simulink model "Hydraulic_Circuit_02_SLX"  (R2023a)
settings: Solver=ode23s  StartTime=0.0  StopTime=10.0  MaxStep=0.001  RelTol=1e-3
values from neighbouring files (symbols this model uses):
  C_5 = 0.001*m^3/Pa    (= 0.001)    [Hydraulic_Circuit_02_EQN.m]    (also in Hydraulic_Circuit_02_SLX_m.m; Electric_Circuit_02_EQN.m; Electric_Circuit_02_SLX_m.m; Electric_Circuit_04_EQN.m)
  C_7 = 0.001*m^3/Pa    (= 0.001)    [Hydraulic_Circuit_02_EQN.m]    (also in Hydraulic_Circuit_02_SLX_m.m; Electric_Circuit_02_EQN.m; Electric_Circuit_02_SLX_m.m; Electric_Circuit_04_EQN.m)
  L_4 = 10*Pa*sec^2/m^3    (= 10)    [Hydraulic_Circuit_02_EQN.m]    (also in Hydraulic_Circuit_02_SLX_m.m; Electric_Circuit_02_EQN.m = 0.002; Electric_Circuit_02_SLX_m.m = 0.002; Electric_Circuit_03_EQN.m = 0.002)
  L_6 = 10*Pa*sec^2/m^3    (= 10)    [Hydraulic_Circuit_02_EQN.m]    (also in Hydraulic_Circuit_02_SLX_m.m; Electric_Circuit_07_EQN.m = 0.002; Electric_Circuit_07_SLX_m.m = 0.002; Hydraulic_Circuit_03_EQN.m)
  P_1_0 = 10*Pa    (= 10)    [Hydraulic_Circuit_02_SLX_m.m]    (also in Hydraulic_Circuit_01_SLX_m.m; Hydraulic_Circuit_03_SLX_m.m; Hydraulic_Clutch_System_SLX_m.m)
  P_5_0 = 0*Pa    (= 0)    [Hydraulic_Circuit_02_SLX_m.m]    (also in Hydraulic_Circuit_03_SLX_m.m)
  P_7_0 = 0*Pa    (= 0)    [Hydraulic_Circuit_02_SLX_m.m]
  Q_4_0 = 0*m^3/sec    (= 0)    [Hydraulic_Circuit_02_SLX_m.m]    (also in Hydraulic_Circuit_03_SLX_m.m)
  Q_6_0 = 0*m^3/sec    (= 0)    [Hydraulic_Circuit_02_SLX_m.m]    (also in Hydraulic_Circuit_03_SLX_m.m)
  Q_9_0 = 0*m^3/sec    (= 0)    [Hydraulic_Circuit_02_SLX_m.m]
  R_2 = 10000*Pa/(m^3/sec)    (= 10000)    [Hydraulic_Circuit_02_EQN.m]    (also in Hydraulic_Circuit_02_SLX_m.m; BIG_EC_Simscape_EQN.m = 100; BIG_EC_Simscape_SLX_m.m = 100; Electric_Circuit_07_EQN.m = 100)
  R_3 = 10000*Pa/(m^3/sec)    (= 10000)    [Hydraulic_Circuit_02_EQN.m]    (also in Hydraulic_Circuit_02_SLX_m.m; Electric_Circuit_01_EQN.m = 100; Electric_Circuit_01_SLX_m.m = 100; Electric_Circuit_02_EQN.m = 100)
  R_8 = 10000*Pa/(m^3/sec)    (= 10000)    [Hydraulic_Circuit_02_EQN.m]    (also in Hydraulic_Circuit_02_SLX_m.m; Electric_Circuit_10_EQN.m = 100; Electric_Circuit_10_SLX_m.m = 100)
  Ts = Tfin/Nr_Ts_Points    (= 0.03999985)    [Hydraulic_Circuit_02_SLX_m.m]    (also in BIG_EC_Simscape_SLX_m.m = 0.0003; Car_Dumper_SLX_m.m = 0.0022779; Electric_Circuit_01_SLX_m.m = 0.005; Electric_Circuit_02_SLX_m.m = 0.000480145)

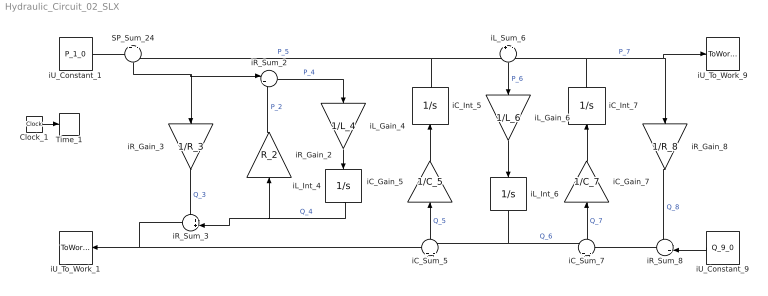
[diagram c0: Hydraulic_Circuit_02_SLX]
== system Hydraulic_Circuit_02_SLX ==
  Clock_1 : Clock
  SP_Sum_24 : Sum  Inputs=+|-
  Time_1 : ToWorkspace  VariableName=t  SaveFormat=Timeseries  SampleTime=Ts
  iC_Gain_5 : Gain  Gain=1/C_5  Multiplication=Matrix(K*u)
  iC_Gain_7 : Gain  Gain=1/C_7  Multiplication=Matrix(K*u)
  iC_Int_5 : Integrator  InitialCondition=P_5_0
  iC_Int_7 : Integrator  InitialCondition=P_7_0
  iC_Sum_5 : Sum  Inputs=+|-
  iC_Sum_7 : Sum  Inputs=+|-
  iL_Gain_4 : Gain  Gain=1/L_4  Multiplication=Matrix(K*u)
  iL_Gain_6 : Gain  Gain=1/L_6  Multiplication=Matrix(K*u)
  iL_Int_4 : Integrator  InitialCondition=Q_4_0
  iL_Int_6 : Integrator  InitialCondition=Q_6_0
  iL_Sum_6 : Sum  Inputs=+|-
  iR_Gain_2 : Gain  Gain=R_2  Multiplication=Matrix(K*u)
  iR_Gain_3 : Gain  Gain=1/R_3  Multiplication=Matrix(K*u)
  iR_Gain_8 : Gain  Gain=1/R_8  Multiplication=Matrix(K*u)
  iR_Sum_2 : Sum  Inputs=|+-
  iR_Sum_3 : Sum  Inputs=++|
  iR_Sum_8 : Sum  Inputs=++|
  iU_Constant_1 : Constant  Value=P_1_0
  iU_Constant_9 : Constant  Value=Q_9_0
  iU_To_Work_1 : ToWorkspace  VariableName=Q_1_0  SaveFormat=Timeseries  SampleTime=Ts
  iU_To_Work_9 : ToWorkspace  VariableName=P_9_0  SaveFormat=Timeseries  SampleTime=Ts
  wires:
  iU_Constant_1/1 -> SP_Sum_24/1
  iC_Int_5/1 -> SP_Sum_24/2, iL_Sum_6/1  "P_5"
  iR_Sum_3/1 -> iU_To_Work_1/1, iC_Sum_5/1
  SP_Sum_24/1 -> iR_Gain_3/1, iR_Sum_2/1
  iL_Int_4/1 -> iR_Sum_3/2, iR_Gain_2/1  "Q_4"
  iR_Gain_3/1 -> iR_Sum_3/1  "Q_3"
  iR_Sum_2/1 -> iL_Gain_4/1  "P_4"
  iR_Gain_2/1 -> iR_Sum_2/2  "P_2"
  iL_Gain_4/1 -> iL_Int_4/1
  iL_Int_6/1 -> iC_Sum_5/2, iC_Sum_7/1  "Q_6"
  iC_Sum_5/1 -> iC_Gain_5/1  "Q_5"
  iC_Gain_5/1 -> iC_Int_5/1
  iC_Int_7/1 -> iL_Sum_6/2, iU_To_Work_9/1, iR_Gain_8/1  "P_7"
  iL_Sum_6/1 -> iL_Gain_6/1  "P_6"
  iL_Gain_6/1 -> iL_Int_6/1
  iR_Sum_8/1 -> iC_Sum_7/2
  iC_Sum_7/1 -> iC_Gain_7/1  "Q_7"
  iC_Gain_7/1 -> iC_Int_7/1
  iU_Constant_9/1 -> iR_Sum_8/2
  iR_Gain_8/1 -> iR_Sum_8/1  "Q_8"
  Clock_1/1 -> Time_1/1
